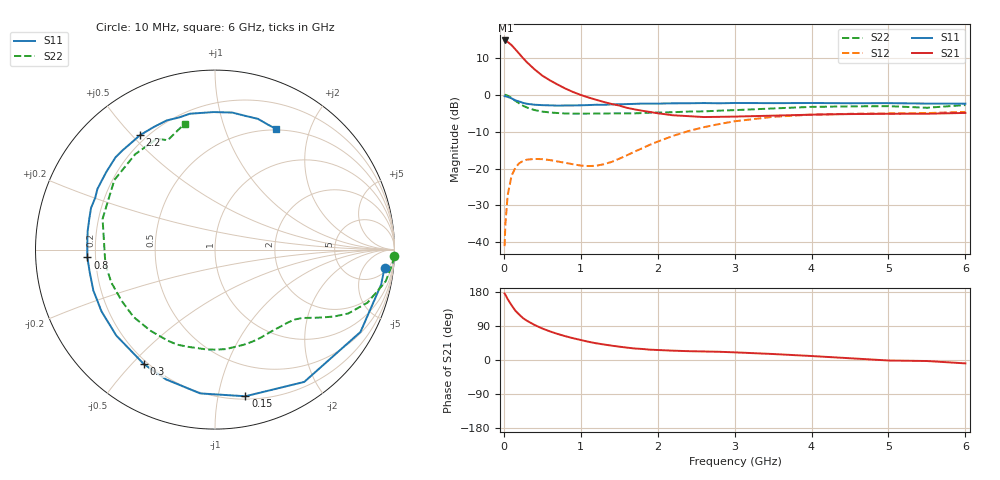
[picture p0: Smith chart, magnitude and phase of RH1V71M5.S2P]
! SIEMENS Small Signal Semiconductors
! BFR106
! Si NPN RF Bipolar Junction Transistor in SOT23
! VCE = 1.75 V  IC = 1.5 mA
! Common Emitter S-Parameters:  August  1996
# GHz  S  MA  R  50
!  f  S11  S21  S12  S22
! GHz  MAG  ANG  MAG  ANG  MAG  ANG  MAG  ANG
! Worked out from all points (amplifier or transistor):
!   36 points, 10 MHz to 6 GHz, reference 50 ohm
!   highest |S21| = 14.6 dB at 20 MHz (marker M1)
!   |S21| within 3 dB of that: start of sweep to 175.1 MHz
!   unconditionally stable (mu >= 1): 805.2 MHz to end of sweep
!   at 250 MHz: K = 0.30, MSG = 13.9 dB, |S12| = -18.0 dB
!   at 1.4 GHz: K = 1.38, MAG = 4.2 dB, |S12| = -18.2 dB
!   at 6 GHz: K = 1.02, MAG = -1.0 dB, |S12| = -4.7 dB
!   S11 on the Smith chart (normalised r, x): 10 MHz: 7, -15; 150 MHz: 0.22, -1.20; 300 MHz: 0.18, -0.54; 800 MHz: 0.17, -0.03; 2.2 GHz: 0.17, +0.53; 6 GHz: 0.48, +1.51
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0.01  0.9502 -6.1  5.396 175.4  0.0089 87.5  0.9985 -2.2
0.02  0.946 -11.9  5.4 172.4  0.0177 82.9  0.9927 -4.4
0.05  0.9314 -29.5  5.155 160.5  0.0438 73.1  0.9674 -10.5
0.1  0.8892 -56.0  4.677 144.6  0.0795 59.4  0.9005 -19.1
0.15  0.8345 -78.3  4.093 130.0  0.1028 47.6  0.8237 -25.6
0.2  0.8055 -95.9  3.573 119.8  0.1179 39.8  0.7615 -29.3
0.25  0.7729 -110.7  3.112 110.4  0.1265 33.1  0.7058 -32.4
0.3  0.7513 -121.8  2.74 103.6  0.1316 28.7  0.6689 -34.6
0.4  0.7292 -139.0  2.19 92.4  0.1348 22.2  0.6173 -38.1
0.5  0.72 -151.4  1.806 83.1  0.1338 18.6  0.589 -41.5
0.6  0.715 -161.5  1.557 75.4  0.13 16.6  0.5735 -45.3
0.8  0.7124 -176.5  1.207 62.8  0.1194 18.1  0.5553 -53.9
1.1  0.7213 166.1  0.914 48.1  0.1079 30.9  0.5534 -68.2
1.6  0.7442 144.5  0.662 32.7  0.1511 58.8  0.5584 -94.6
2.2  0.7622 123.2  0.525 24.6  0.2766 60.3  0.5775 -128.5
2.8  0.7629 105.3  0.5 21.7  0.3997 47.7  0.6061 -162.4
3.5  0.7663 90.5  0.519 15.8  0.5001 31.0  0.6494 164.7
4  0.7695 82.8  0.535 10.5  0.536 20.2  0.6819 145.3
4.5  0.764 77.0  0.545 4.6  0.5497 11.1  0.6928 129.9
5  0.7667 71.8  0.55 -1.3  0.5566 3.8  0.6976 117.6
5.5  0.7557 66.7  0.551 -2.7  0.5623 0.5  0.6638 113.4
6  0.7538 63.4  0.565 -8.9  0.5831 -7.0  0.7213 103.6
